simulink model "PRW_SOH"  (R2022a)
settings: Solver=FixedStepAuto  StartTime=0.0  StopTime=770000  FixedStep=1  RelTol=1e-3
undefined symbols (not defined in the file or in its folder): D, dSOC_mu_PRW, dSOC_sig_PRW, dv_mu_PRW, dv_sig_PRW, PRW_LSTM_Network, PRW_model_only_SOH, S280406_Matlab_Script, SOC_mu_PRW, SOC_sig_PRW, SOE_mu_PRW, SOE_sig_PRW, Thesis
libraries: deeplib x1

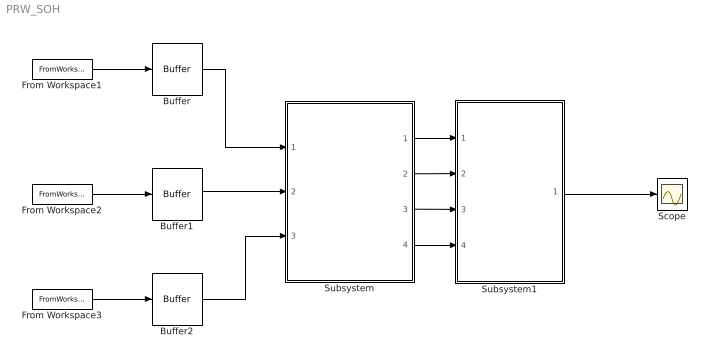
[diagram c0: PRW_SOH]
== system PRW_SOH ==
  Buffer : Buffer  N=120  OutputFrames=off
  Buffer1 : Buffer  N=120  OutputFrames=off
  Buffer2 : Buffer  N=120  OutputFrames=off
  From Workspace1 : FromWorkspace  VariableName=Voltage_03  SampleTime=1
  From Workspace2 : FromWorkspace  VariableName=Current_03  SampleTime=1
  From Workspace3 : FromWorkspace  VariableName=SOC  SampleTime=1
  Scope : Scope
  Subsystem : Subsystem
  Subsystem1 : Subsystem
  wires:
  Buffer2/1 -> Subsystem/3(SOC_03)
  From Workspace3/1 -> Buffer2/1
  Subsystem/1(dSOC) -> Subsystem1/1(dSOC)
  Subsystem/2(dV) -> Subsystem1/2(dv)
  From Workspace1/1 -> Buffer/1
  From Workspace2/1 -> Buffer1/1
  Buffer1/1 -> Subsystem/2(I_03)
  Buffer/1 -> Subsystem/1(V_03)
  Subsystem1/1(Input1) -> Scope/1
  Subsystem/3(SOC) -> Subsystem1/3(SOC)
  Subsystem/4(SOE) -> Subsystem1/4(SOE)

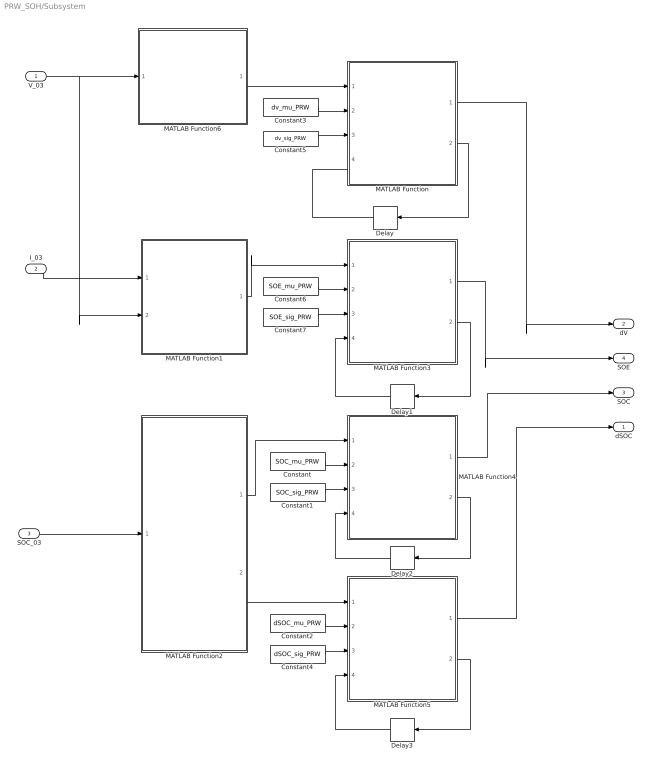
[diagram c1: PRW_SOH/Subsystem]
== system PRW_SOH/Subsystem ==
  V_03 : Inport
  I_03 : Inport  Port=2
  SOC_03 : Inport  Port=3
  Constant : Constant  Value=SOC_mu_PRW
  Constant1 : Constant  Value=SOC_sig_PRW
  Constant2 : Constant  Value=dSOC_mu_PRW
  Constant3 : Constant  Value=dv_mu_PRW
  Constant4 : Constant  Value=dSOC_sig_PRW
  Constant5 : Constant  Value=dv_sig_PRW
  Constant6 : Constant  Value=SOE_mu_PRW
  Constant7 : Constant  Value=SOE_sig_PRW
  Delay{,1..3} (4 alike) : Delay  DelayLength=1
  MATLAB Function : MATLAB Function  TreatAsAtomicUnit=on
  MATLAB Function1 : MATLAB Function  TreatAsAtomicUnit=on
  MATLAB Function2 : MATLAB Function  TreatAsAtomicUnit=on
  MATLAB Function3 : MATLAB Function  TreatAsAtomicUnit=on
  MATLAB Function4 : MATLAB Function  TreatAsAtomicUnit=on
  MATLAB Function5 : MATLAB Function  TreatAsAtomicUnit=on
  MATLAB Function6 : MATLAB Function  TreatAsAtomicUnit=on
  dSOC : Outport
  dV : Outport  Port=2
  SOC : Outport  Port=3
  SOE : Outport  Port=4
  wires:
  Constant5/1 -> MATLAB Function/3(dv_sig_CC)
  Constant3/1 -> MATLAB Function/2(dv_mu_CC)
  V_03/1 -> MATLAB Function1/2(V_03), MATLAB Function6/1(V_03)
  I_03/1 -> MATLAB Function1/1(I_03)
  SOC_03/1 -> MATLAB Function2/1(SOC_03)
  Delay/1 -> MATLAB Function/4(dv_previous_tmp)
  MATLAB Function/2(dv) -> Delay/1
  MATLAB Function/1(dv_filt) -> dV/1
  Delay1/1 -> MATLAB Function3/4(SOE_previous_tmp)
  Constant7/1 -> MATLAB Function3/3(SOE_sig_CC)
  MATLAB Function3/1(SOE_filt) -> SOE/1
  Constant6/1 -> MATLAB Function3/2(SOE_mu_CC)
  MATLAB Function3/2(SOE) -> Delay1/1
  MATLAB Function1/1(SOE) -> MATLAB Function3/1("SOE ")
  Constant1/1 -> MATLAB Function4/3(SOC_sig_CC)
  MATLAB Function4/2(SOC) -> Delay2/1
  MATLAB Function4/1(SOC_filt) -> SOC/1
  MATLAB Function2/1(SOC) -> MATLAB Function4/1("SOC ")
  Constant/1 -> MATLAB Function4/2(SOC_mu_CC)
  Delay2/1 -> MATLAB Function4/4(SOC_previous_tmp)
  Constant2/1 -> MATLAB Function5/2(dSOC_mu_CC)
  Delay3/1 -> MATLAB Function5/4(dSOC_previous_tmp)
  Constant4/1 -> MATLAB Function5/3(dSOC_sig_CC)
  MATLAB Function2/2(dSOC) -> MATLAB Function5/1("dSOC ")
  MATLAB Function5/2(dSOC) -> Delay3/1
  MATLAB Function5/1(dSOC_filt) -> dSOC/1
  MATLAB Function6/1(dv) -> MATLAB Function/1("dv ")

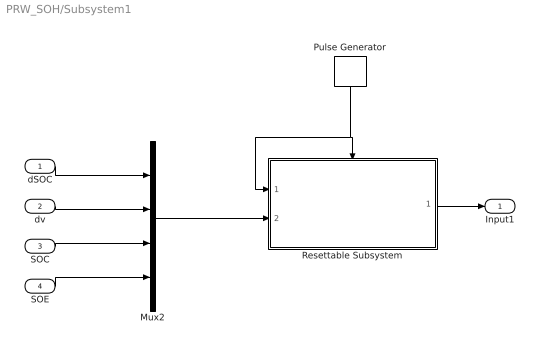
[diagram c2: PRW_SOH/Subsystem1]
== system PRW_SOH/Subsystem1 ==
  dSOC : Inport
  dv : Inport  Port=2
  SOC : Inport  Port=3
  SOE : Inport  Port=4
  Mux2 : Mux
  Pulse Generator : DiscretePulseGenerator  PulseType=Time based  Period=120  PulseWidth=1/120*100  PhaseDelay=119
  Resettable Subsystem : Subsystem  TreatAsAtomicUnit=on
  Input1 : Outport
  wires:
  Mux2/1 -> Resettable Subsystem/2(Input1)
  dSOC/1 -> Mux2/1
  dv/1 -> Mux2/2
  SOC/1 -> Mux2/3
  SOE/1 -> Mux2/4
  Pulse Generator/1 -> Resettable Subsystem/1(Input), Resettable Subsystem/Reset
  Resettable Subsystem/1(Out1) -> Input1/1

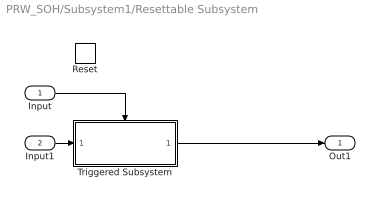
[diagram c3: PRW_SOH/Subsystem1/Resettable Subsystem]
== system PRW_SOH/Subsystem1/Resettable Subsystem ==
  Input : Inport
  Input1 : Inport  Port=2
  Reset : ResetPort  DisableCoverage=on
  Triggered Subsystem : Subsystem  TreatAsAtomicUnit=on
  Out1 : Outport
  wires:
  Triggered Subsystem/1(Out1) -> Out1/1
  Input/1 -> Triggered Subsystem/Trigger
  Input1/1 -> Triggered Subsystem/1(u)

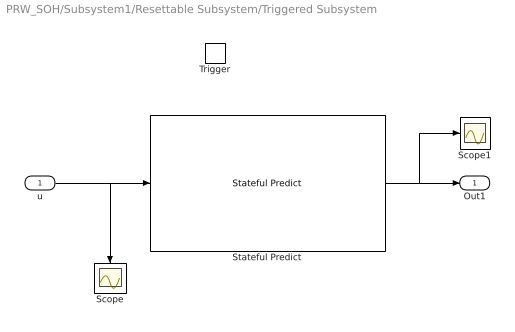
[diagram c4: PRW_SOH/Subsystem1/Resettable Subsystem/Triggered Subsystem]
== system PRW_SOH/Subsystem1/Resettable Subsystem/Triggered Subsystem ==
  u : Inport
  Trigger : TriggerPort  TriggerType=falling  VariantControl=(inherit)
  Scope : Scope
  Scope1 : Scope
  Stateful Predict : deeplib/Stateful Predict  Network=Network from MAT-file  NetworkFunction=untitled  NetworkFilePath=D:\Thesis\S280406_Matlab_Script\PRW_model_only_SOH\PRW_LSTM_Network.mat  InputDataFormats={ '', '' }  SampleTime=-1  ForceInterpretedSim=off  EnableDLNetwork=on
  Out1 : Outport
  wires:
  u/1 -> Stateful Predict/1, Scope/1
  Stateful Predict/1 -> Scope1/1, Out1/1

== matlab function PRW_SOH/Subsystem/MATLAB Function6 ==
function dv = fcn(V_03)
dv = V_03(120)-V_03(1);
end

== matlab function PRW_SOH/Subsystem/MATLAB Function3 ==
function [SOE_filt, SOE]  = SOE_filter(SOE,SOE_mu_CC,SOE_sig_CC,SOE_previous_tmp)

persistent SOE_previous

if isempty(SOE_previous)
    SOE_previous = 0;
else
    SOE_previous = [SOE_previous , SOE_previous_tmp];
end

[b,a]=butter(1,0.000001);
SOE_filt_tmp = (filter(b,a,[SOE_previous SOE],[],2)-SOE_mu_CC)./SOE_sig_CC;
SOE_filt = SOE_filt_tmp(end);

end

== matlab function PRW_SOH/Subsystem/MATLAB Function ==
function [dv_filt, dv]  = dv_filter(dv,dv_mu_CC,dv_sig_CC,dv_previous_tmp)

persistent dv_previous

if isempty(dv_previous)
    dv_previous = 0;
else
    dv_previous = [dv_previous , dv_previous_tmp];
end


[b,a]=butter(1,0.000001);
dv_filt_tmp = (filter(b,a,[dv_previous dv],[],2)-dv_mu_CC)./dv_sig_CC;
dv_filt = dv_filt_tmp(end);

end

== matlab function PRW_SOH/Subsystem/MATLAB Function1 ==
function SOE  = SOE(I_03,V_03)

persistent  E1 E2 E3 E4 dE flag1 flag2 count SOE_reg
if isempty(E1)
    E1 = 0;
    E2 = 0;
    E3 = 0;
    E4 = 0;
    dE = 0;
    flag1 = 0;
    flag2 = 1;
    count = 0;
    SOE_reg = 0;
end

if I_03 ~= 0
    count = count+1;
end

if I_03(1)~=0 && flag1 ==0 && flag2 == 1
    E1 = I_03(1)*V_03(1);
    E2 = I_03(120)*V_03(120);
    flag1 = 1;
    flag2 = 0;
elseif I_03(1)~=0 && flag1 == 1 && flag2 == 0
    E3 = I_03(1)*V_03(1);
    E4 = I_03(120)*V_03(120);
    flag1 = 0;
    flag2 = 1;
end

SOE1 = zeros(1,120);

if count == 1
    SOE1(1) = 0;
elseif mod(count,2) == 1
    dE = (E1-E4)/2;
    SOE1(1) = SOE_reg+dE;
else
    dE = (E3-E2)/2;
    SOE1(1) = SOE_reg+dE;
end

time = linspace(1,120,120);
E = I_03.*V_03;
SOE_cum = cumtrapz(time,E);
k = 2;

for i = 1:119
    SOE1(k) = SOE_cum(i+1)-SOE_cum(i);
    k = k+1;
end

SOE_reg = SOE1(120);

SOE = SOE1(120);

end

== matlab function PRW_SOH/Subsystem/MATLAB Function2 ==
function [SOC,dSOC] = SOC_features(SOC_03)
SOC = SOC_03(120);

dSOC = SOC_03(120)-SOC_03(1);

if dSOC<-10
    dSOC = 0;
end
end

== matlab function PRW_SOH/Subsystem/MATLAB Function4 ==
function [SOC_filt, SOC]  = SOC_filter(SOC,SOC_mu_CC,SOC_sig_CC,SOC_previous_tmp)

persistent SOC_previous

if isempty(SOC_previous)
    SOC_previous = 0;
else
    SOC_previous = [SOC_previous , SOC_previous_tmp];
end

[b,a]=butter(1,0.000001);
SOC_filt_tmp = (filter(b,a,[SOC_previous SOC],[],2)-SOC_mu_CC)./SOC_sig_CC;
SOC_filt = SOC_filt_tmp(end);

end

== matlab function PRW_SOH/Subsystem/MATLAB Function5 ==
function [dSOC_filt, dSOC]  = dSOC_filter(dSOC,dSOC_mu_CC,dSOC_sig_CC,dSOC_previous_tmp)

persistent dSOC_previous

if isempty(dSOC_previous)
    dSOC_previous = 0;
else
    dSOC_previous = [dSOC_previous , dSOC_previous_tmp];
end

[b,a]=butter(1,0.000001);
dSOC_filt_tmp = (filter(b,a,[dSOC_previous dSOC],[],2)-dSOC_mu_CC)./dSOC_sig_CC;
dSOC_filt = dSOC_filt_tmp(end);

end
